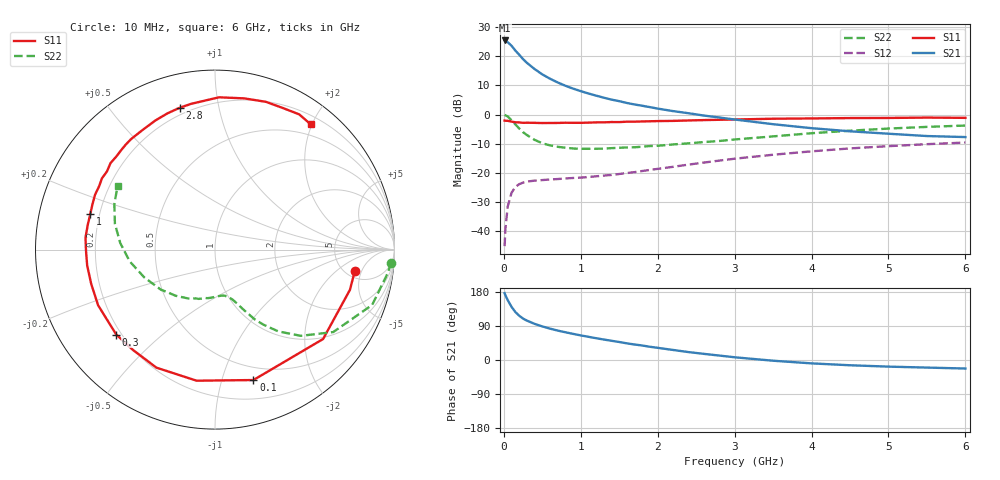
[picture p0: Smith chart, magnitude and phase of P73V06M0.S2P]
! SIEMENS Small Signal Semiconductors
! BFP196
! Si NPN RF Bipolar Junction Transistor in SOT143
! VCE = 3 V  IC = 6 mA
! Common Emitter S-Parameters:  May  1996
# GHz  S  MA  R  50
!  f  S11  S21  S12  S22
! GHz  MAG  ANG  MAG  ANG  MAG  ANG  MAG  ANG
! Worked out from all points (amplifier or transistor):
!   36 points, 10 MHz to 6 GHz, reference 50 ohm
!   highest |S21| = 25.4 dB at 10 MHz (marker M1)
!   |S21| within 3 dB of that: start of sweep to 136.2 MHz
!   unconditionally stable (mu >= 1): 1.031 GHz to 3.172 GHz
!   at 250 MHz: K = 0.29, MSG = 21.1 dB, |S12| = -23.3 dB
!   at 1.4 GHz: K = 1.15, MAG = 10.5 dB, |S12| = -20.7 dB
!   at 6 GHz: K = 1.00, MSG = 0.9 dB, |S12| = -9.6 dB
!   S11 on the Smith chart (normalised r, x): 10 MHz: 6.09, -3.75; 100 MHz: 0.37, -1.27; 300 MHz: 0.18, -0.36; 1 GHz: 0.16, +0.14; 2.8 GHz: 0.16, +0.77; 6 GHz: 0.32, +1.98
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0.01  0.7882 -8.5  18.53 176.5  0.0056 86.0  0.9847 -4.2
0.02  0.7846 -16.6  18.06 170.8  0.0109 85.0  0.9707 -7.9
0.05  0.7816 -39.6  17.32 158.2  0.0266 70.3  0.9282 -19.4
0.1  0.7576 -73.6  15.06 140.3  0.0459 55.9  0.8031 -34.9
0.15  0.7376 -98.0  12.44 126.5  0.0577 44.7  0.6782 -45.1
0.2  0.7342 -116.4  10.56 116.8  0.0645 37.6  0.5772 -52.2
0.25  0.7223 -129.5  8.882 109.3  0.0685 32.8  0.4987 -57.1
0.3  0.7257 -139.3  7.668 103.9  0.0714 30.3  0.4462 -60.4
0.4  0.7214 -154.5  6.006 95.4  0.074 26.4  0.3691 -64.7
0.5  0.7157 -164.5  4.867 88.6  0.0757 25.0  0.3231 -67.9
0.6  0.7177 -172.9  4.108 82.8  0.0775 24.9  0.2968 -70.5
0.8  0.7247 174.7  3.112 73.2  0.0807 25.5  0.2704 -75.5
1  0.7225 164.0  2.514 64.9  0.0833 27.9  0.2592 -80.9
1.1  0.7278 159.8  2.293 61.2  0.0855 29.5  0.2594 -83.8
1.3  0.7357 151.4  1.942 54.0  0.0904 32.2  0.2615 -89.6
1.6  0.7557 140.4  1.577 43.9  0.0999 35.9  0.2737 -98.7
2.2  0.7792 121.1  1.146 26.5  0.1277 40.0  0.3083 -117.3
2.8  0.8142 104.0  0.891 11.7  0.163 38.9  0.3532 -137.3
3.5  0.8488 88.5  0.684 -1.9  0.2054 33.1  0.4232 -158.5
4.5  0.8708 71.0  0.517 -13.9  0.2636 22.0  0.5293 176.0
5.5  0.8875 58.1  0.429 -20.0  0.3114 9.9  0.6154 155.7
6  0.8782 52.6  0.412 -22.5  0.3321 3.3  0.6486 146.8
